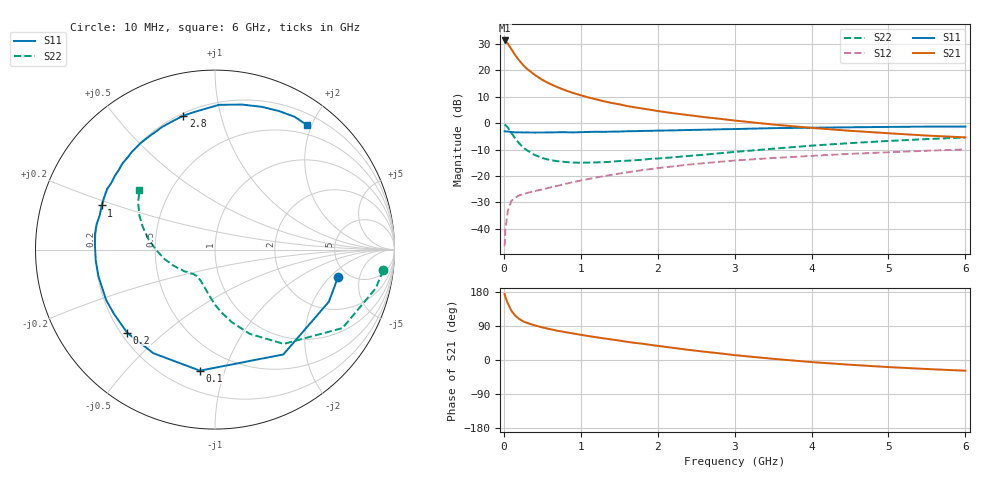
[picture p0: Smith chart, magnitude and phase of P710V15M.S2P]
! SIEMENS Small Signal Semiconductors
! BFP196
! Si NPN RF Bipolar Junction Transistor in SOT143
! VCE = 10 V  IC = 15 mA
! Common Emitter S-Parameters:  May  1996
# GHz  S  MA  R  50
!  f  S11  S21  S12  S22
! GHz  MAG  ANG  MAG  ANG  MAG  ANG  MAG  ANG
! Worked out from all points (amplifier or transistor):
!   36 points, 10 MHz to 6 GHz, reference 50 ohm
!   highest |S21| = 31.3 dB at 10 MHz (marker M1)
!   |S21| within 3 dB of that: start of sweep to 91.64 MHz
!   unconditionally stable (mu >= 1): 823.8 MHz to 3.487 GHz
!   at 250 MHz: K = 0.49, MSG = 24.5 dB, |S12| = -26.9 dB
!   at 1.4 GHz: K = 1.12, MAG = 11.5 dB, |S12| = -19.6 dB
!   at 6 GHz: K = 0.96, MSG = 2.3 dB, |S12| = -9.9 dB
!   S11 on the Smith chart (normalised r, x): 10 MHz: 4.16, -2.50; 100 MHz: 0.33, -0.83; 200 MHz: 0.22, -0.38; 1 GHz: 0.20, +0.18; 2.8 GHz: 0.21, +0.77; 6 GHz: 0.36, +1.94
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0.01  0.7027 -12.5  36.89 173.9  0.0047 83.0  0.944 -7.0
0.02  0.6977 -24.6  35.64 166.5  0.0096 74.0  0.9214 -13.5
0.05  0.6973 -56.9  32.24 149.9  0.0215 62.7  0.8342 -31.6
0.1  0.6798 -97.1  25.03 129.4  0.0341 49.1  0.6503 -53.9
0.15  0.6718 -120.8  19.18 116.6  0.0391 42.0  0.5077 -67.6
0.2  0.6739 -136.6  15.44 108.3  0.043 39.1  0.4147 -77.0
0.25  0.6671 -147.7  12.64 102.2  0.0453 37.7  0.3479 -84.6
0.3  0.6685 -155.1  10.76 98.0  0.0477 37.6  0.3077 -89.9
0.4  0.6662 -167.0  8.248 91.4  0.0519 38.2  0.251 -98.4
0.5  0.6672 -174.8  6.634 86.1  0.0557 40.4  0.2189 -105.2
0.6  0.6689 178.4  5.56 81.4  0.0606 42.1  0.2012 -110.6
0.7  0.6743 172.8  4.798 77.1  0.0655 43.9  0.1906 -114.9
0.8  0.6748 168.1  4.195 73.5  0.0711 45.0  0.1844 -118.8
1  0.6773 158.7  3.377 66.5  0.0821 46.5  0.1787 -124.6
1.1  0.683 154.6  3.079 63.2  0.0878 47.2  0.18 -127.6
1.6  0.7044 137.0  2.117 48.1  0.1171 46.4  0.1952 -139.1
2.2  0.7312 119.0  1.547 32.1  0.1525 42.4  0.2263 -151.1
2.8  0.7669 103.3  1.216 17.7  0.1857 36.3  0.2693 -165.5
3.5  0.8069 88.4  0.945 3.1  0.2193 28.4  0.3292 -179.9
4.5  0.8372 71.8  0.719 -12.5  0.2628 17.7  0.4199 162.9
5.5  0.8626 59.1  0.583 -23.8  0.3015 7.1  0.501 148.7
6  0.8628 53.4  0.54 -28.3  0.3195 1.3  0.5362 141.8
